| Texas Instruments Incorporated
| Low Additive Jitter LVDS buffers
| Marketing part#  Voltage Range   Pkg-type  #pins/pkg   Inputs/Outputs
| LMK1D1208   1.71V-3.465V   QFN   28-pin QFN   2:8
| LMK1D1204   1.71V-3.465V   QFN   16-pin QFN   2:4
| LMK1D2104   1.71V-3.465V   QFN   28-pin QFN   Dual 1:4
| LMK1D2102   1.71V-3.465V   QFN   16-pin QFN   Dual 1:2
| LMK1D1204P   1.71V-3.465V   QFN   28-pin QFN   2:4 w/ output ctrl
| LMK1D1216   1.71V-3.465V   QFN   48-pin QFN   2:16
| LMK1D1212   1.71V-3.465V   QFN   40-pin QFN   2:12
| LMK1D2108   1.71V-3.465V   QFN   48-pin QFN   Dual 1:8
| LMK1D2106   1.71V-3.465V   QFN   40-pin QFN   Dual 1:6
| LMK1D1208I   1.71V-3.465V   QFN   40-pin QFN   2:8 w/ I2C ctrl
| LMK1D1208P   1.71V-3.465V   QFN   40-pin QFN   2:8 w/ output ctrl
[IBIS Ver] 4.1
[File name] lmk1dxx_w_hs.ibs
[File Rev] 1.1
[Date] 11/18/2022
[Source]
| Texas Instruments Incorporated.
| 12500 TI Blvd
| Dallas, TX -75243
[Notes] Revision History:
| Rev 1.1: 11/18/2022
| -  Added Rac and Cac parameters to the LVDS_OUT models
|   -  These parameters cause an error flag in IBIS checker, but have been
|   validated against SPECTRE simulations for better accuracy
|   -  These Rac/Cac parameters may be commented-out, but can result in unrealistic
|   large reflections in the output signal
| Rev 1.0: 10/11/2021
| - Initial version of the model
| - Model generated from simulations in SPECTRE
| - C_comp although listed in numerical order of value are
| obtained from varying PVT conditions. For PVT conditions for
| each specific value refer the buffer description under
| respective [Model]. IBIS model user is responsible for using
| appropriate C_comp to simulate for Signal Integrity.
| - Warnings regarding combined Non-monotonicity of various models have been
| reviewed and considered minor and can be ignored.
|| - Model names with a trailing _1P8 contain the model for
| 1.8V operation. Model names with a trailing _2P5or3P3 contain the model
| for 2.5V or 3.3V operation. Model names with a trailing _HS contain the model
| for high-swing outputs, if supported by that Component
[Disclaimer]
| This model is designed as an aid for customers of Texas Instruments.
| TI and its licensors and suppliers make no warranties, either expressed
| or implied, with respect to this model, including the warranties of
| merchantability or fitness for a particular purpose. The model is
| provided solely on an "as is" basis. The entire risk as to its quality
| and performance is with the customer.
| This model is subject to change without notice. Texas Instruments
| Incorporated is not responsible for updating this model.
[Copyright]
(C) Copyright 2021 Texas Instruments Incorporated. All rights reserved.
| Component LMK1D1208
[Component] LMK1D1208
[Manufacturer] Texas Instruments Incorporated
[Package] |QFN (RHD) 28-pin
| variable typ min max
R_pkg 0.12 0.1 0.141
L_pkg 1.3nH 1.2nH 1.55nH
C_pkg 0.25pF 0.2pF 0.3pF
| pin number (pin name) mapping to model name
[Pin]   signal_name   model_name   R_pin   L_pin   C_pin
1   GND   GND   0.0660  1.46858n   0.24532p
2   OUT7_P   LVDS_OUT   0.1208  1.3245n   0.21958p
3   OUT7_N   LVDS_OUT   0.1120  1.23426n   0.20877p
4   IN_SEL   TRI_IN   0.1104  1.22239n   0.204p
5   IN1_P   LVDS_IN   0.1140  1.25533n   0.21096p
6   IN1_N   LVDS_IN   0.1252  1.37778n   0.2223p
7   VAC_REF1   NC   0.1367  1.50244n   0.20733p
8   VDD   POWER   0.0502  1.4703n   0.30681p
9   IN0_P   LVDS_IN   0.1235  1.35569n   0.22656p
10   IN0_N   LVDS_IN   0.1147  1.26942n   0.21367p
11   VAC_REF0   NC   0.1137  1.26025n   0.20504p
12   OUT0_P   LVDS_OUT   0.1167  1.28716n   0.2115p
13   OUT0_N   LVDS_OUT   0.1272  1.39578n   0.22776p
14   GND   GND   0.0697  1.52734n   0.26393p
15   VDD   POWER   0.0666  1.54716n   0.26564p
16   OUT1_P   LVDS_OUT   0.1210  1.32692n   0.21617p
17   OUT1_N   LVDS_OUT   0.1118  1.23394n   0.20744p
18   OUT2_P   LVDS_OUT   0.1101  1.21502n   0.20318p
19   OUT2_N   LVDS_OUT   0.1143  1.26234n   0.20922p
20   OUT3_P   LVDS_OUT   0.1218  1.34856n   0.21848p
21   OUT3_N   LVDS_OUT   0.1373  1.50472n   0.20606p
22   OUT4_P   LVDS_OUT   0.1414  1.5481n   0.21484p
23   OUT4_N   LVDS_OUT   0.1269  1.39145n   0.22511p
24   OUT5_P   LVDS_OUT   0.1165  1.2851n   0.21442p
25   OUT5_N   LVDS_OUT   0.1134  1.25105n   0.20643p
26   OUT6_P   LVDS_OUT   0.1152  1.27172n   0.2105p
27   OUT6_N   LVDS_OUT   0.1236  1.36371n   0.2247p
28   VDD   POWER   0.0676  1.4842n   0.25361p
| Differential pin definition
[Diff Pin] inv_pin vdiff tdelay_typ tdelay_min tdelay_max
| The 'OUTx_P' pin is Diff_pin and the 'OUTx_N' pin is the inv_pin
| The 'INx_P' pin is Diff_pin and the 'INx_N' pin is the inv_pin
2   3   0.200   0 0 0
5   6   0.200   0 0 0
9   10   0.200   0 0 0
12   13   0.200   0 0 0
16   17   0.200   0 0 0
18   19   0.200   0 0 0
20   21   0.200   0 0 0
22   23   0.200   0 0 0
24   25   0.200   0 0 0
26   27   0.200   0 0 0
|***** end of component 1 definition
| Component2 LMK1D1204
[Component] LMK1D1204
[Manufacturer] Texas Instruments Incorporated
[Package] |QFN (RGT) 16-pin
| variable typ min max
R_pkg 0.07 0.06 0.10
L_pkg 0.8nH 0.68nH 1.11nH
C_pkg 0.15pF 0.12pF 0.18pF
| pin number (pin name) mapping to model name
[Pin]   signal_name   model_name   R_pin   L_pin   C_pin
1   GND   GND   0.0341  0.7311n   0.12954p
2   IN_SEL   TRI_IN   0.0667  0.68218n   0.13512p
3   IN1_P   LVDS_IN   0.0702  0.72664n   0.14532p
4   IN1_N   LVDS_IN   0.0867  0.926n   0.14036p
5   VDD   POWER   0.027   0.83n   0.18251p
6   IN0_P   LVDS_IN   0.0763  0.80494n   0.15746p
7   IN0_N   LVDS_IN   0.0855  0.90879n   0.16432p
8   VAC_REF   NC   0.1026  1.11478n   0.15521p
9   OUT0_P   LVDS_OUT   0.0802  0.85219n   0.13221p
10   OUT0_N   LVDS_OUT   0.0679  0.69177n   0.143p
11   OUT1_P   LVDS_OUT   0.0676  0.68903n   0.14122p
12   OUT1_N   LVDS_OUT   0.0701  0.72841n   0.12345p
13   OUT2_P   LVDS_OUT   0.0717  0.75236n   0.12274p
14   OUT2_N   LVDS_OUT   0.0629  0.63165n   0.13417p
15   OUT3_P   LVDS_OUT   0.0631  0.62827n   0.13463p
16   OUT3_N   LVDS_OUT   0.0728  0.75998n   0.1242p
| Differential pin definition
[Diff Pin] inv_pin vdiff tdelay_typ tdelay_min tdelay_max
| The 'OUTx_P' pin is Diff_pin and the 'OUTx_N' pin is the inv_pin
| The 'INx_P' pin is Diff_pin and the 'INx_N' pin is the inv_pin
3   4   0.200   0 0 0
6   7   0.200   0 0 0
9   10   0.200   0 0 0
11   12   0.200   0 0 0
13   14   0.200   0 0 0
15   16   0.200   0 0 0
|***** end of component 2 definition
| Component3 LMK1D2104
[Component] LMK1D2104
[Manufacturer] Texas Instruments Incorporated
[Package] |QFN (RHD) 28-pin
| variable typ min max
R_pkg 0.12 0.1 0.141
L_pkg 1.3nH 1.2nH 1.55nH
C_pkg 0.25pF 0.2pF 0.3pF
| pin number (pin name) mapping to model name
[Pin]   signal_name   model_name   R_pin   L_pin   C_pin
1   GND   GND   0.0660  1.46858n   0.24532p
2   OUT7_P   LVDS_OUT   0.1208  1.3245n   0.21958p
3   OUT7_N   LVDS_OUT   0.1120  1.23426n   0.20877p
4   EN   TRI_IN   0.1104  1.22239n   0.204p
5   IN1_P   LVDS_IN   0.1140  1.25533n   0.21096p
6   IN1_N   LVDS_IN   0.1252  1.37778n   0.2223p
7   VAC_REF1   NC   0.1367  1.50244n   0.20733p
8   VDD   POWER   0.0502  1.4703n   0.30681p
9   IN0_P   LVDS_IN   0.1235  1.35569n   0.22656p
10   IN0_N   LVDS_IN   0.1147  1.26942n   0.21367p
11   VAC_REF0   NC   0.1137  1.26025n   0.20504p
12   OUT0_P   LVDS_OUT   0.1167  1.28716n   0.2115p
13   OUT0_N   LVDS_OUT   0.1272  1.39578n   0.22776p
14   GND   GND   0.0697  1.52734n   0.26393p
15   VDD   POWER   0.0666  1.54716n   0.26564p
16   OUT1_P   LVDS_OUT   0.1210  1.32692n   0.21617p
17   OUT1_N   LVDS_OUT   0.1118  1.23394n   0.20744p
18   OUT2_P   LVDS_OUT   0.1101  1.21502n   0.20318p
19   OUT2_N   LVDS_OUT   0.1143  1.26234n   0.20922p
20   OUT3_P   LVDS_OUT   0.1218  1.34856n   0.21848p
21   OUT3_N   LVDS_OUT   0.1373  1.50472n   0.20606p
22   OUT4_P   LVDS_OUT   0.1414  1.5481n   0.21484p
23   OUT4_N   LVDS_OUT   0.1269  1.39145n   0.22511p
24   OUT5_P   LVDS_OUT   0.1165  1.2851n   0.21442p
25   OUT5_N   LVDS_OUT   0.1134  1.25105n   0.20643p
26   OUT6_P   LVDS_OUT   0.1152  1.27172n   0.2105p
27   OUT6_N   LVDS_OUT   0.1236  1.36371n   0.2247p
28   VDD   POWER   0.0676  1.4842n   0.25361p
| Differential pin definition
[Diff Pin] inv_pin vdiff tdelay_typ tdelay_min tdelay_max
| The 'OUTx_P' pin is Diff_pin and the 'OUTx_N' pin is the inv_pin
| The 'INx_P' pin is Diff_pin and the 'INx_N' pin is the inv_pin
2   3   0.200   0 0 0
5   6   0.200   0 0 0
9   10   0.200   0 0 0
12   13   0.200   0 0 0
16   17   0.200   0 0 0
18   19   0.200   0 0 0
20   21   0.200   0 0 0
22   23   0.200   0 0 0
24   25   0.200   0 0 0
26   27   0.200   0 0 0
|***** end of component 3 definition
| Component4 LMK1D2102
[Component] LMK1D2102
[Manufacturer] Texas Instruments Incorporated
[Package] |QFN (RGT) 16-pin
| variable typ min max
R_pkg 0.07 0.06 0.10
L_pkg 0.8nH 0.68nH 1.11nH
C_pkg 0.15pF 0.12pF 0.18pF
| pin number (pin name) mapping to model name
[Pin]   signal_name   model_name   R_pin   L_pin   C_pin
1   GND   GND   0.0341  0.7311n   0.12954p
2   EN   TRI_IN   0.0667  0.68218n   0.13512p
3   IN1_P   LVDS_IN   0.0702  0.72664n   0.14532p
4   IN1_N   LVDS_IN   0.0867  0.926n   0.14036p
5   VDD   POWER   0.027   0.83n   0.18251p
6   IN0_P   LVDS_IN   0.0763  0.80494n   0.15746p
7   IN0_N   LVDS_IN   0.0855  0.90879n   0.16432p
8   VAC_REF   NC   0.1026  1.11478n   0.15521p
9   OUT0_P   LVDS_OUT   0.0802  0.85219n   0.13221p
10   OUT0_N   LVDS_OUT   0.0679  0.69177n   0.143p
11   OUT1_P   LVDS_OUT   0.0676  0.68903n   0.14122p
12   OUT1_N   LVDS_OUT   0.0701  0.72841n   0.12345p
13   OUT2_P   LVDS_OUT   0.0717  0.75236n   0.12274p
14   OUT2_N   LVDS_OUT   0.0629  0.63165n   0.13417p
15   OUT3_P   LVDS_OUT   0.0631  0.62827n   0.13463p
16   OUT3_N   LVDS_OUT   0.0728  0.75998n   0.1242p
| Differential pin definition
[Diff Pin] inv_pin vdiff tdelay_typ tdelay_min tdelay_max
| The 'OUTx_P' pin is Diff_pin and the 'OUTx_N' pin is the inv_pin
| The 'INx_P' pin is Diff_pin and the 'INx_N' pin is the inv_pin
3   4   0.200   0 0 0
6   7   0.200   0 0 0
9   10   0.200   0 0 0
11   12   0.200   0 0 0
13   14   0.200   0 0 0
15   16   0.200   0 0 0
|***** end of component 4 definition
| Component5 LMK1D1204P
[Component] LMK1D1204P
[Manufacturer] Texas Instruments Incorporated
[Package] |QFN (RHD) 28-pin
| variable typ min max
R_pkg 0.12 0.1 0.141
L_pkg 1.3nH 1.2nH 1.55nH
C_pkg 0.25pF 0.2pF 0.3pF
| pin number (pin name) mapping to model name
[Pin]   signal_name   model_name   R_pin   L_pin   C_pin
1   GND   GND   0.0660  1.46858n   0.24532p
2   IN_SEL   TRI_IN   0.1208  1.3245n   0.21958p
3   OE3   I2C_IN   0.1120  1.23426n   0.20877p
4   NC   NC   NA   NA   NA
5   IN1_P   LVDS_IN   0.1140  1.25533n   0.21096p
6   IN1_N   LVDS_IN   0.1252  1.37778n   0.2223p
7   VAC_REF1   NC   0.1367  1.50244n   0.20733p
8   VDD   POWER   0.0502  1.4703n   0.30681p
9   IN0_P   LVDS_IN   0.1235  1.35569n   0.22656p
10   IN0_N   LVDS_IN   0.1147  1.26942n   0.21367p
11   VAC_REF0   NC   0.1137  1.26025n   0.20504p
12   NC   NC   NA   NA   NA
13   OE0   I2C_IN   0.1272  1.39578n   0.22776p
14   GND   GND   0.0697  1.52734n   0.26393p
15   VDD   POWER   0.0666  1.54716n   0.26564p
16   OUT0_P   LVDS_OUT   0.1210  1.32692n   0.21617p
17   OUT0_N   LVDS_OUT   0.1118  1.23394n   0.20744p
18   NC   NC   NA   NA   NA
19   OE1   I2C_IN   0.1143  1.26234n   0.20922p
20   OUT1_P   LVDS_OUT   0.1218  1.34856n   0.21848p
21   OUT1_N   LVDS_OUT   0.1373  1.50472n   0.20606p
22   OUT2_P   LVDS_OUT   0.1414  1.5481n   0.21484p
23   OUT2_N   LVDS_OUT   0.1269  1.39145n   0.22511p
24   OE2   I2C_IN   0.1165  1.2851n   0.21442p
25   NC   NC   NA   NA   NA
26   OUT3_P   LVDS_OUT   0.1152  1.27172n   0.2105p
27   OUT3_N   LVDS_OUT   0.1236  1.36371n   0.2247p
28   VDD   POWER   0.0676  1.4842n   0.25361p
| Differential pin definition
[Diff Pin] inv_pin vdiff tdelay_typ tdelay_min tdelay_max
| The 'OUTx_P' pin is Diff_pin and the 'OUTx_N' pin is the inv_pin
| The 'INx_P' pin is Diff_pin and the 'INx_N' pin is the inv_pin
2   3   0.200   0 0 0
5   6   0.200   0 0 0
9   10   0.200   0 0 0
12   13   0.200   0 0 0
16   17   0.200   0 0 0
18   19   0.200   0 0 0
20   21   0.200   0 0 0
22   23   0.200   0 0 0
24   25   0.200   0 0 0
26   27   0.200   0 0 0
|***** end of component 5 definition
|   Component LMK1D1216
[Component]   LMK1D1216
[Manufacturer] Texas Instruments Incorporated
[Package]   |QFN (RGZ) 48-pin
|   typ   min   max
R_pkg   0.11   0.10   0.14
L_pkg   1.65nH   1.47nH   1.92nH
C_pkg   0.24pF   0.21pF   0.30pF
[Pin]   signal_name   model_name   R_pin   L_pin   C_pin
1   GND   GND   0.0637  1.34721n   0.28801p
2   IN_SEL   TRI_IN   0.11858 1.74642n   0.25783p
3   IN1_P   LVDS_IN   0.11074 1.62917n   0.24222p
4   IN1_N   LVDS_IN   0.10483 1.54045n   0.23511p
5   VAC_REF1   NC   0.1013  1.48833n   0.22312p
6   VDD   POWER   0.1004  1.4784n   0.21502p
7   VDD   POWER   0.10067 1.4833n   0.21361p
8   VAC_REF0   NC   0.1012  1.48775n   0.22167p
9   IN0_N   LVDS_IN   0.10463 1.54219n   0.23426p
10   IN0_P   LVDS_IN   0.11042 1.64325n   0.23372p
11   AMP_SEL   TRI_IN   0.11042 1.64325n   0.23372p
12   GND   GND   0.06347 1.36215n   0.2136p
13   VDD   POWER   0.06559 1.38685n   0.27375p
14   OUT0_P   LVDS_OUT   0.12562 1.85789n   0.28633p
15   OUT0_N   LVDS_OUT   0.11759 1.73367n   0.25978p
16   OUT1_P   LVDS_OUT   0.11132 1.6387n   0.24963p
17   OUT1_N   LVDS_OUT   0.1072  1.57642n   0.24106p
18   OUT2_P   LVDS_OUT   0.10558 1.55335n   0.23421p
19   OUT2_N   LVDS_OUT   0.10652 1.5673n   0.22874p
20   OUT3_P   LVDS_OUT   0.10983 1.6171n   0.2299p
21   OUT3_N   LVDS_OUT   0.11552 1.70685n   0.23544p
22   OUT4_P   LVDS_OUT   0.11542 1.6983n   0.23814p
23   OUT4_N   LVDS_OUT   0.12293 1.80466n   0.2402p
24   VDD   POWER   0.06573 1.37071n   0.26233p
25   OUT5_P   LVDS_OUT   0.13288 1.91697n   0.29383p
26   OUT5_N   LVDS_OUT   0.12185 1.77242n   0.25417p
27   OUT6_P   LVDS_OUT   0.11341 1.65363n   0.26077p
28   OUT6_N   LVDS_OUT   0.10674 1.56205n   0.24554p
29   OUT7_P   LVDS_OUT   0.10228 1.50028n   0.23778p
30   OUT7_N   LVDS_OUT   0.10042 1.47685n   0.22809p
31   OUT8_P   LVDS_OUT   0.10038 1.47619n   0.21747p
32   OUT8_N   LVDS_OUT   0.102   1.49553n   0.21725p
33   OUT9_P   LVDS_OUT   0.10625 1.55482n   0.22778p
34   OUT9_N   LVDS_OUT   0.11272 1.64361n   0.23744p
35   OUT10_P   LVDS_OUT   0.12102 1.75951n   0.24504p
36   OUT10_N   LVDS_OUT   0.13192 1.90158n   0.25953p
37   VDD   POWER   0.06574 1.36809n   0.25297p
38   OUT11_P   LVDS_OUT   0.12292 1.80433n   0.29418p
39   OUT11_N   LVDS_OUT   0.11542 1.69805n   0.26222p
40   OUT12_P   LVDS_OUT   0.11551 1.70689n   0.2401p
41   OUT12_N   LVDS_OUT   0.10983 1.61712n   0.23799p
42   OUT13_P   LVDS_OUT   0.10652 1.56806n   0.23512p
43   OUT13_N   LVDS_OUT   0.10559 1.55307n   0.23015p
44   OUT14_P   LVDS_OUT   0.10721 1.57701n   0.22876p
45   OUT14_N   LVDS_OUT   0.11131 1.63895n   0.23439p
46   OUT15_P   LVDS_OUT   0.11758 1.73438n   0.24099p
47   OUT15_N   LVDS_OUT   0.12561 1.858n   0.24976p
48   VDD   POWER   0.06559 1.38505n   0.25978p
[Diff_pin]   inv_pin   vdiff   tdelay_typ   tdelay_min   tdelay_max
| The 'OUTx_P' pin is Diff_pin and the 'OUTx_N' pin is the inv_pin
| The 'INx_P' pin is Diff_pin and the 'INx_N' pin is the inv_pin
3   4   0.200   0   0   0
9   10   0.200   0   0   0
14   15   0.200   0   0   0
16   17   0.200   0   0   0
18   19   0.200   0   0   0
20   21   0.200   0   0   0
22   23   0.200   0   0   0
25   26   0.200   0   0   0
27   28   0.200   0   0   0
29   30   0.200   0   0   0
31   32   0.200   0   0   0
33   34   0.200   0   0   0
35   36   0.200   0   0   0
38   39   0.200   0   0   0
40   41   0.200   0   0   0
42   43   0.200   0   0   0
44   45   0.200   0   0   0
46   47   0.200   0   0   0
|***** end of component 6 definition
|   Component7 LMK1D1212
[Component]   LMK1D1212
[Manufacturer]  Texas Instruments Incorporated
[Package]   |QFN (RHA) 40-pin
|   typ   min   max
R_pkg   0.126   0.077   0.155
L_pkg   1.91nH   1.64nH   2.26nH
C_pkg   0.215pF   0.196pF   0.239pF
[Pin]   signal_name   model_name   R_pin   L_pin   C_pin
1   IN_SEL   TRI_IN   0.15532 2.25319n   0.21485p
2   IN1_P   LVDS_IN   0.13841 2.05109n   0.23658p
3   IN1_N   LVDS_IN   0.12544 1.86801n   0.21892p
4   VAC_REF1   NC   0.11676 1.73939n   0.20751p
5   VDD   POWER   0.11607 1.74363n   0.20235p
6   VDD   POWER   0.11342 1.70024n   0.20454p
7   VAC_REF0   NC   0.1166  1.74464n   0.20682p
8   IN0_N   LVDS_IN   0.12513 1.86484n   0.21917p
9   IN0_P   LVDS_IN   0.13798 2.04129n   0.23931p
10   AMP_SEL   TRI_IN   0.15481 2.24016n   0.21648p
11   VDD   POWER   0.07699 1.64721n   0.2394p
12   OUT0_P   LVDS_OUT   0.14237 2.13276n   0.21831p
13   OUT0_N   LVDS_OUT   0.12994 1.94924n   0.22306p
14   OUT1_P   LVDS_OUT   0.12176 1.827n   0.21156p
15   OUT1_N   LVDS_OUT   0.1187  1.7845n   0.20484p
16   OUT2_P   LVDS_OUT   0.11945 1.7986n   0.20452p
17   OUT2_N   LVDS_OUT   0.1249  1.88587n   0.21258p
18   OUT3_P   LVDS_OUT   0.12793 1.92595n   0.21417p
19   OUT3_N   LVDS_OUT   0.13959 2.09594n   0.22416p
20   VDD   POWER   0.07715 1.67594n   0.24728p
21   GND   GND   0.0753  1.64217n   0.24086p
22   OUT4_P   LVDS_OUT   0.13548 2.03086n   0.23377p
23   OUT4_N   LVDS_OUT   0.12329 1.84977n   0.21506p
24   OUT5_P   LVDS_OUT   0.11566 1.73691n   0.20666p
25   OUT5_N   LVDS_OUT   0.11347 1.71236n   0.19605p
26   OUT6_P   LVDS_OUT   0.11353 1.71348n   0.19848p
27   OUT6_N   LVDS_OUT   0.11537 1.73371n   0.20693p
28   OUT7_P   LVDS_OUT   0.1227  1.84205n   0.2154p
29   OUT7_N   LVDS_OUT   0.13466 2.01897n   0.23649p
30   GND   GND   0.07482 1.62936n   0.24263p
31   VDD   POWER   0.07715 1.67476n   0.24579p
32   OUT8_P   LVDS_OUT   0.1396  2.09565n   0.2202p
33   OUT8_N   LVDS_OUT   0.12793 1.92612n   0.2152p
34   OUT9_P   LVDS_OUT   0.12491 1.88517n   0.20914p
35   OUT9_N   LVDS_OUT   0.11945 1.79917n   0.20553p
36   OUT10_P   LVDS_OUT   0.11869 1.78536n   0.20479p
37   OUT10_N   LVDS_OUT   0.12174 1.82891n   0.21303p
38   OUT11_P   LVDS_OUT   0.12994 1.95074n   0.22296p
39   OUT11_N   LVDS_OUT   0.14237 2.13405n   0.2213p
40   VDD   POWER   0.07699 1.64783n   0.23928p
[Diff_pin]   inv_pin   vdiff   tdelay_typ   tdelay_min   tdelay_max
| The 'OUTx_P' pin is Diff_pin and the 'OUTx_N' pin is the inv_pin
| The 'INx_P' pin is Diff_pin and the 'INx_N' pin is the inv_pin
2   3   0.200   0 0 0
8   9   0.200   0 0 0
12   13   0.200   0 0 0
14   15   0.200   0 0 0
16   17   0.200   0 0 0
18   19   0.200   0 0 0
22   23   0.200   0 0 0
24   25   0.200   0 0 0
26   27   0.200   0 0 0
28   29   0.200   0 0 0
32   33   0.200   0 0 0
34   35   0.200   0 0 0
36   37   0.200   0 0 0
38   39   0.200   0 0 0
|***** end of component 7 definition
|   Component LMK1D2108
[Component]   LMK1D2108
[Manufacturer]  Texas Instruments Incorporated
[Package]   |QFN (RGZ) 48-pin
|   typ   min   max
R_pkg   0.11   0.10   0.14
L_pkg   1.65nH   1.47nH   1.92nH
C_pkg   0.24pF   0.21pF   0.30pF
[Pin]   signal_name   model_name   R_pin   L_pin   C_pin
1   GND   GND   0.0637  1.34721n   0.28801p
2   EN   TRI_IN   0.11858 1.74642n   0.25783p
3   IN1_P   LVDS_IN   0.11074 1.62917n   0.24222p
4   IN1_N   LVDS_IN   0.10483 1.54045n   0.23511p
5   VAC_REF1   NC   0.1013  1.48833n   0.22312p
6   VDD   POWER   0.1004  1.4784n   0.21502p
7   VDD   POWER   0.10067 1.4833n   0.21361p
8   VAC_REF0   NC   0.1012  1.48775n   0.22167p
9   IN0_N   LVDS_IN   0.10463 1.54219n   0.23426p
10   IN0_P   LVDS_IN   0.11042 1.64325n   0.23372p
11   AMP_SEL   TRI_IN   0.11042 1.64325n   0.23372p
12   GND   GND   0.06347 1.36215n   0.2136p
13   VDD   POWER   0.06559 1.38685n   0.27375p
14   OUT0_P   LVDS_OUT   0.12562 1.85789n   0.28633p
15   OUT0_N   LVDS_OUT   0.11759 1.73367n   0.25978p
16   OUT1_P   LVDS_OUT   0.11132 1.6387n   0.24963p
17   OUT1_N   LVDS_OUT   0.1072  1.57642n   0.24106p
18   OUT2_P   LVDS_OUT   0.10558 1.55335n   0.23421p
19   OUT2_N   LVDS_OUT   0.10652 1.5673n   0.22874p
20   OUT3_P   LVDS_OUT   0.10983 1.6171n   0.2299p
21   OUT3_N   LVDS_OUT   0.11552 1.70685n   0.23544p
22   OUT4_P   LVDS_OUT   0.11542 1.6983n   0.23814p
23   OUT4_N   LVDS_OUT   0.12293 1.80466n   0.2402p
24   VDD   POWER   0.06573 1.37071n   0.26233p
25   OUT5_P   LVDS_OUT   0.13288 1.91697n   0.29383p
26   OUT5_N   LVDS_OUT   0.12185 1.77242n   0.25417p
27   OUT6_P   LVDS_OUT   0.11341 1.65363n   0.26077p
28   OUT6_N   LVDS_OUT   0.10674 1.56205n   0.24554p
29   OUT7_P   LVDS_OUT   0.10228 1.50028n   0.23778p
30   OUT7_N   LVDS_OUT   0.10042 1.47685n   0.22809p
31   OUT8_P   LVDS_OUT   0.10038 1.47619n   0.21747p
32   OUT8_N   LVDS_OUT   0.102   1.49553n   0.21725p
33   OUT9_P   LVDS_OUT   0.10625 1.55482n   0.22778p
34   OUT9_N   LVDS_OUT   0.11272 1.64361n   0.23744p
35   OUT10_P   LVDS_OUT   0.12102 1.75951n   0.24504p
36   OUT10_N   LVDS_OUT   0.13192 1.90158n   0.25953p
37   VDD   POWER   0.06574 1.36809n   0.25297p
38   OUT11_P   LVDS_OUT   0.12292 1.80433n   0.29418p
39   OUT11_N   LVDS_OUT   0.11542 1.69805n   0.26222p
40   OUT12_P   LVDS_OUT   0.11551 1.70689n   0.2401p
41   OUT12_N   LVDS_OUT   0.10983 1.61712n   0.23799p
42   OUT13_P   LVDS_OUT   0.10652 1.56806n   0.23512p
43   OUT13_N   LVDS_OUT   0.10559 1.55307n   0.23015p
44   OUT14_P   LVDS_OUT   0.10721 1.57701n   0.22876p
45   OUT14_N   LVDS_OUT   0.11131 1.63895n   0.23439p
46   OUT15_P   LVDS_OUT   0.11758 1.73438n   0.24099p
47   OUT15_N   LVDS_OUT   0.12561 1.858n   0.24976p
48   VDD   POWER   0.06559 1.38505n   0.25978p
[Diff_pin]   inv_pin   vdiff   tdelay_typ   tdelay_min   tdelay_max
| The 'OUTx_P' pin is Diff_pin and the 'OUTx_N' pin is the inv_pin
| The 'INx_P' pin is Diff_pin and the 'INx_N' pin is the inv_pin
3   4   0.200   0   0   0
9   10   0.200   0   0   0
14   15   0.200   0   0   0
16   17   0.200   0   0   0
18   19   0.200   0   0   0
20   21   0.200   0   0   0
22   23   0.200   0   0   0
25   26   0.200   0   0   0
27   28   0.200   0   0   0
29   30   0.200   0   0   0
31   32   0.200   0   0   0
33   34   0.200   0   0   0
35   36   0.200   0   0   0
38   39   0.200   0   0   0
40   41   0.200   0   0   0
42   43   0.200   0   0   0
44   45   0.200   0   0   0
46   47   0.200   0   0   0
|***** end of component 6 definition
|   Component9 LMK1D2106
[Component]   LMK1D2106
[Manufacturer]  Texas Instruments Incorporated
[Package]   |QFN (RHA) 40-pin
|   typ   min   max
R_pkg   0.126   0.077   0.155
L_pkg   1.91nH   1.64nH   2.26nH
C_pkg   0.215pF   0.196pF   0.239pF
[Pin]   signal_name   model_name   R_pin   L_pin   C_pin
1   EN   TRI_IN   0.15532 2.25319n   0.21485p
2   IN1_P   LVDS_IN   0.13841 2.05109n   0.23658p
3   IN1_N   LVDS_IN   0.12544 1.86801n   0.21892p
4   VAC_REF1   NC   0.11676 1.73939n   0.20751p
5   VDD   POWER   0.11607 1.74363n   0.20235p
6   VDD   POWER   0.11342 1.70024n   0.20454p
7   VAC_REF0   NC   0.1166  1.74464n   0.20682p
8   IN0_N   LVDS_IN   0.12513 1.86484n   0.21917p
9   IN0_P   LVDS_IN   0.13798 2.04129n   0.23931p
10   AMP_SEL   TRI_IN   0.15481 2.24016n   0.21648p
11   VDD   POWER   0.07699 1.64721n   0.2394p
12   OUT0_P   LVDS_OUT   0.14237 2.13276n   0.21831p
13   OUT0_N   LVDS_OUT   0.12994 1.94924n   0.22306p
14   OUT1_P   LVDS_OUT   0.12176 1.827n   0.21156p
15   OUT1_N   LVDS_OUT   0.1187  1.7845n   0.20484p
16   OUT2_P   LVDS_OUT   0.11945 1.7986n   0.20452p
17   OUT2_N   LVDS_OUT   0.1249  1.88587n   0.21258p
18   OUT3_P   LVDS_OUT   0.12793 1.92595n   0.21417p
19   OUT3_N   LVDS_OUT   0.13959 2.09594n   0.22416p
20   VDD   POWER   0.07715 1.67594n   0.24728p
21   GND   GND   0.0753  1.64217n   0.24086p
22   OUT4_P   LVDS_OUT   0.13548 2.03086n   0.23377p
23   OUT4_N   LVDS_OUT   0.12329 1.84977n   0.21506p
24   OUT5_P   LVDS_OUT   0.11566 1.73691n   0.20666p
25   OUT5_N   LVDS_OUT   0.11347 1.71236n   0.19605p
26   OUT6_P   LVDS_OUT   0.11353 1.71348n   0.19848p
27   OUT6_N   LVDS_OUT   0.11537 1.73371n   0.20693p
28   OUT7_P   LVDS_OUT   0.1227  1.84205n   0.2154p
29   OUT7_N   LVDS_OUT   0.13466 2.01897n   0.23649p
30   GND   GND   0.07482 1.62936n   0.24263p
31   VDD   POWER   0.07715 1.67476n   0.24579p
32   OUT8_P   LVDS_OUT   0.1396  2.09565n   0.2202p
33   OUT8_N   LVDS_OUT   0.12793 1.92612n   0.2152p
34   OUT9_P   LVDS_OUT   0.12491 1.88517n   0.20914p
35   OUT9_N   LVDS_OUT   0.11945 1.79917n   0.20553p
36   OUT10_P   LVDS_OUT   0.11869 1.78536n   0.20479p
37   OUT10_N   LVDS_OUT   0.12174 1.82891n   0.21303p
38   OUT11_P   LVDS_OUT   0.12994 1.95074n   0.22296p
39   OUT11_N   LVDS_OUT   0.14237 2.13405n   0.2213p
40   VDD   POWER   0.07699 1.64783n   0.23928p
[Diff_pin]   inv_pin   vdiff   tdelay_typ   tdelay_min   tdelay_max
| The 'OUTx_P' pin is Diff_pin and the 'OUTx_N' pin is the inv_pin
| The 'INx_P' pin is Diff_pin and the 'INx_N' pin is the inv_pin
2   3   0.200   0 0 0
8   9   0.200   0 0 0
12   13   0.200   0 0 0
14   15   0.200   0 0 0
16   17   0.200   0 0 0
18   19   0.200   0 0 0
22   23   0.200   0 0 0
24   25   0.200   0 0 0
26   27   0.200   0 0 0
28   29   0.200   0 0 0
32   33   0.200   0 0 0
34   35   0.200   0 0 0
36   37   0.200   0 0 0
38   39   0.200   0 0 0
|***** end of component 9 definition
|   Component LMK1D1208I
[Component]   LMK1D1208I
[Manufacturer]  Texas Instruments Incorporated
[Package]   |QFN (RHA) 40-pin
|   typ   min   max
R_pkg   0.126   0.077   0.155
L_pkg   1.91nH   1.64nH   2.26nH
C_pkg   0.215pF   0.196pF   0.239pF
[Pin]   signal_name   model_name   R_pin   L_pin   C_pin
1   NC   NC   NA   NA   NA
2   OUT7_P   LVDS_OUT   0.13841 2.05109n   0.23658p
3   OUT7N   LVDS_OUT   0.12544 1.86801n   0.21892p
4   NC   NC   NA   NA   NA
5   SDA   I2C_IO   0.11607 1.74363n   0.20235p
6   SCL   I2C_IN   0.11342 1.70024n   0.20454p
7   NC   NC   NA   NA   NA
8   IN1_P   LVDS_IN   0.12513 1.86484n   0.21917p
9   IN1_N   LVDS_IN   0.13798 2.04129n   0.23931p
10   VAC_REF1   NC   0.15481 2.24016n   0.21648p
11   VDD   POWER   0.07699 1.64721n   0.2394p
12   IN0_P   LVDS_IN   0.14237 2.13276n   0.21831p
13   IN0_N   LVDS_IN   0.12994 1.94924n   0.22306p
14   VAC_REF0   NC   0.12176 1.827n   0.21156p
15   IDX0   TRI_IN   0.1187  1.7845n   0.20484p
16   IDX1   TRI_IN   0.11945 1.7986n   0.20452p
17   NC   NC   NA   NA   NA
18   OUT0_P   LVDS_OUT   0.12793 1.92595n   0.21417p
19   OUT0_N   LVDS_OUT   0.13959 2.09594n   0.22416p
20   VDD   POWER   0.07715 1.67594n   0.24728p
21   NC   NC   NA   NA   NA
22   OUT1_P   LVDS_OUT   0.13548 2.03086n   0.23377p
23   OUT1_N   LVDS_OUT   0.12329 1.84977n   0.21506p
24   OUT2_P   LVDS_OUT   0.11566 1.73691n   0.20666p
25   OUT2_N   LVDS_OUT   0.11347 1.71236n   0.19605p
26   NC   NC   NA   NA   NA
27   NC   NC   NA   NA   NA
28   OUT3_P   LVDS_OUT   0.1227  1.84205n   0.2154p
29   OUT3_N   LVDS_OUT   0.13466 2.01897n   0.23649p
30   NC   NC   NA   NA   NA
31   NC   NC   NA   NA   NA
32   OUT4_P   LVDS_OUT   0.1396  2.09565n   0.2202p
33   OUT4_N   LVDS_OUT   0.12793 1.92612n   0.2152p
34   OUT5_P   LVDS_OUT   0.12491 1.88517n   0.20914p
35   OUT5_N   LVDS_OUT   0.11945 1.79917n   0.20553p
36   OUT6_P   LVDS_OUT   0.11869 1.78536n   0.20479p
37   OUT6_N   LVDS_OUT   0.12174 1.82891n   0.21303p
38   OUT7_P   LVDS_OUT   0.12994 1.95074n   0.22296p
39   OUT7_N   LVDS_OUT   0.14237 2.13405n   0.2213p
40   VDD   POWER   0.07699 1.64783n   0.23928p
[Diff_pin]   inv_pin   vdiff   tdelay_typ   tdelay_min   tdelay_max
| The 'OUTx_P' pin is Diff_pin and the 'OUTx_N' pin is the inv_pin
| The 'INx_P' pin is Diff_pin and the 'INx_N' pin is the inv_pin
2   3   0.200   0 0 0
8   9   0.200   0 0 0
12   13   0.200   0 0 0
18   19   0.200   0 0 0
22   23   0.200   0 0 0
24   25   0.200   0 0 0
28   29   0.200   0 0 0
32   33   0.200   0 0 0
34   35   0.200   0 0 0
38   39   0.200   0 0 0
|***** end of component 10 definition
|   Component LMK1D1208P
[Component]   LMK1D1208P
[Manufacturer]  Texas Instruments Incorporated
[Package]   |QFN (RHA) 40-pin
|   typ   min   max
R_pkg   0.126   0.077   0.155
L_pkg   1.91nH   1.64nH   2.26nH
C_pkg   0.215pF   0.196pF   0.239pF
[Pin]   signal_name   model_name   R_pin   L_pin   C_pin
1   IN_SEL   TRI_IN   0.15532 2.25319n   0.21485p
2   IN1_P   LVDS_IN   0.13841 2.05109n   0.23658p
3   IN1_N   LVDS_IN   0.12544 1.86801n   0.21892p
4   VAC_REF1   NC   0.11676 1.73939n   0.20751p
5   OE7   I2C_IN   0.11607 1.74363n   0.20235p
6   OE0   I2C_IN   0.11342 1.70024n   0.20454p
7   VAC_REF0   NC   0.1166  1.74464n   0.20682p
8   IN0_N   LVDS_IN   0.12513 1.86484n   0.21917p
9   IN0_P   LVDS_IN   0.13798 2.04129n   0.23931p
10   AMP_SEL   TRI_IN   0.15481 2.24016n   0.21648p
11   VDD   POWER   0.07699 1.64721n   0.2394p
12   OUT0_P   LVDS_OUT   0.14237 2.13276n   0.21831p
13   OUT0_N   LVDS_OUT   0.12994 1.94924n   0.22306p
14   OUT1_P   LVDS_OUT   0.12176 1.827n   0.21156p
15   OUT1_N   LVDS_OUT   0.1187  1.7845n   0.20484p
16   OE1   I2C_IN   0.11945 1.7986n   0.20452p
17   OE2   I2C_IN   0.1249  1.88587n   0.21258p
18   OE3   I2C_IN   0.12793 1.92595n   0.21417p
19   NC   NC   NA   NA   NA
20   VDD   POWER   0.07715 1.67594n   0.24728p
21   GND   GND   0.0753  1.64217n   0.24086p
22   OUT2_P   LVDS_OUT   0.13548 2.03086n   0.23377p
23   OUT2_N   LVDS_OUT   0.12329 1.84977n   0.21506p
24   OUT3_P   LVDS_OUT   0.11566 1.73691n   0.20666p
25   OUT3_N   LVDS_OUT   0.11347 1.71236n   0.19605p
26   OUT4_P   LVDS_OUT   0.11353 1.71348n   0.19848p
27   OUT4_N   LVDS_OUT   0.11537 1.73371n   0.20693p
28   OUT5_P   LVDS_OUT   0.1227  1.84205n   0.2154p
29   OUT5_N   LVDS_OUT   0.13466 2.01897n   0.23649p
30   GND   GND   0.07482 1.62936n   0.24263p
31   VDD   POWER   0.07715 1.67476n   0.24579p
32   NC   NC   NA   NA   NA
33   OE4   I2C_IN   0.12793 1.92612n   0.2152p
34   OE5   I2C_IN   0.12491 1.88517n   0.20914p
35   OE6   I2C_IN   0.11945 1.79917n   0.20553p
36   OUT6_P   LVDS_OUT   0.11869 1.78536n   0.20479p
37   OUT6_N   LVDS_OUT   0.12174 1.82891n   0.21303p
38   OUT7_P   LVDS_OUT   0.12994 1.95074n   0.22296p
39   OUT7_N   LVDS_OUT   0.14237 2.13405n   0.2213p
40   VDD   POWER   0.07699 1.64783n   0.23928p
[Diff_pin]   inv_pin   vdiff   tdelay_typ   tdelay_min   tdelay_max
| The 'OUTx_P' pin is Diff_pin and the 'OUTx_N' pin is the inv_pin
| The 'INx_P' pin is Diff_pin and the 'INx_N' pin is the inv_pin
2   3   0.200   0 0 0
8   9   0.200   0 0 0
12   13   0.200   0 0 0
14   15   0.200   0 0 0
22   23   0.200   0 0 0
24   25   0.200   0 0 0
26   27   0.200   0 0 0
28   29   0.200   0 0 0
36   37   0.200   0 0 0
38   39   0.200   0 0 0
|***** end of component 11 definition
| Model Selectors
[Model Selector] LVDS_OUT
LVDS_OUT_1P8 LVDS buffer at 1.8V operation.
LVDS_OUT_1P8_HS LVDS buffer at 1.8V operation, in high-swing mode
LVDS_OUT_2P5or3P3 LVDS buffer at 2.5/3.3V operation
LVDS_OUT_2P5or3P3_HS LVDS buffer at 2.5/3.3V operation, in high-swing mode
| Models and submodels in the file (8): LVDS_IN (Input), LVDS_OUT_1P8 (Output), LVDS_OUT_1P8_HS (Output), LVDS_OUT_2P5or3P3 (Output), LVDS_OUT_2P5or3P3_HS (Output), TRI_IN (Input), I2C_IN (Input), I2C_IO (I/O_open_drain)
